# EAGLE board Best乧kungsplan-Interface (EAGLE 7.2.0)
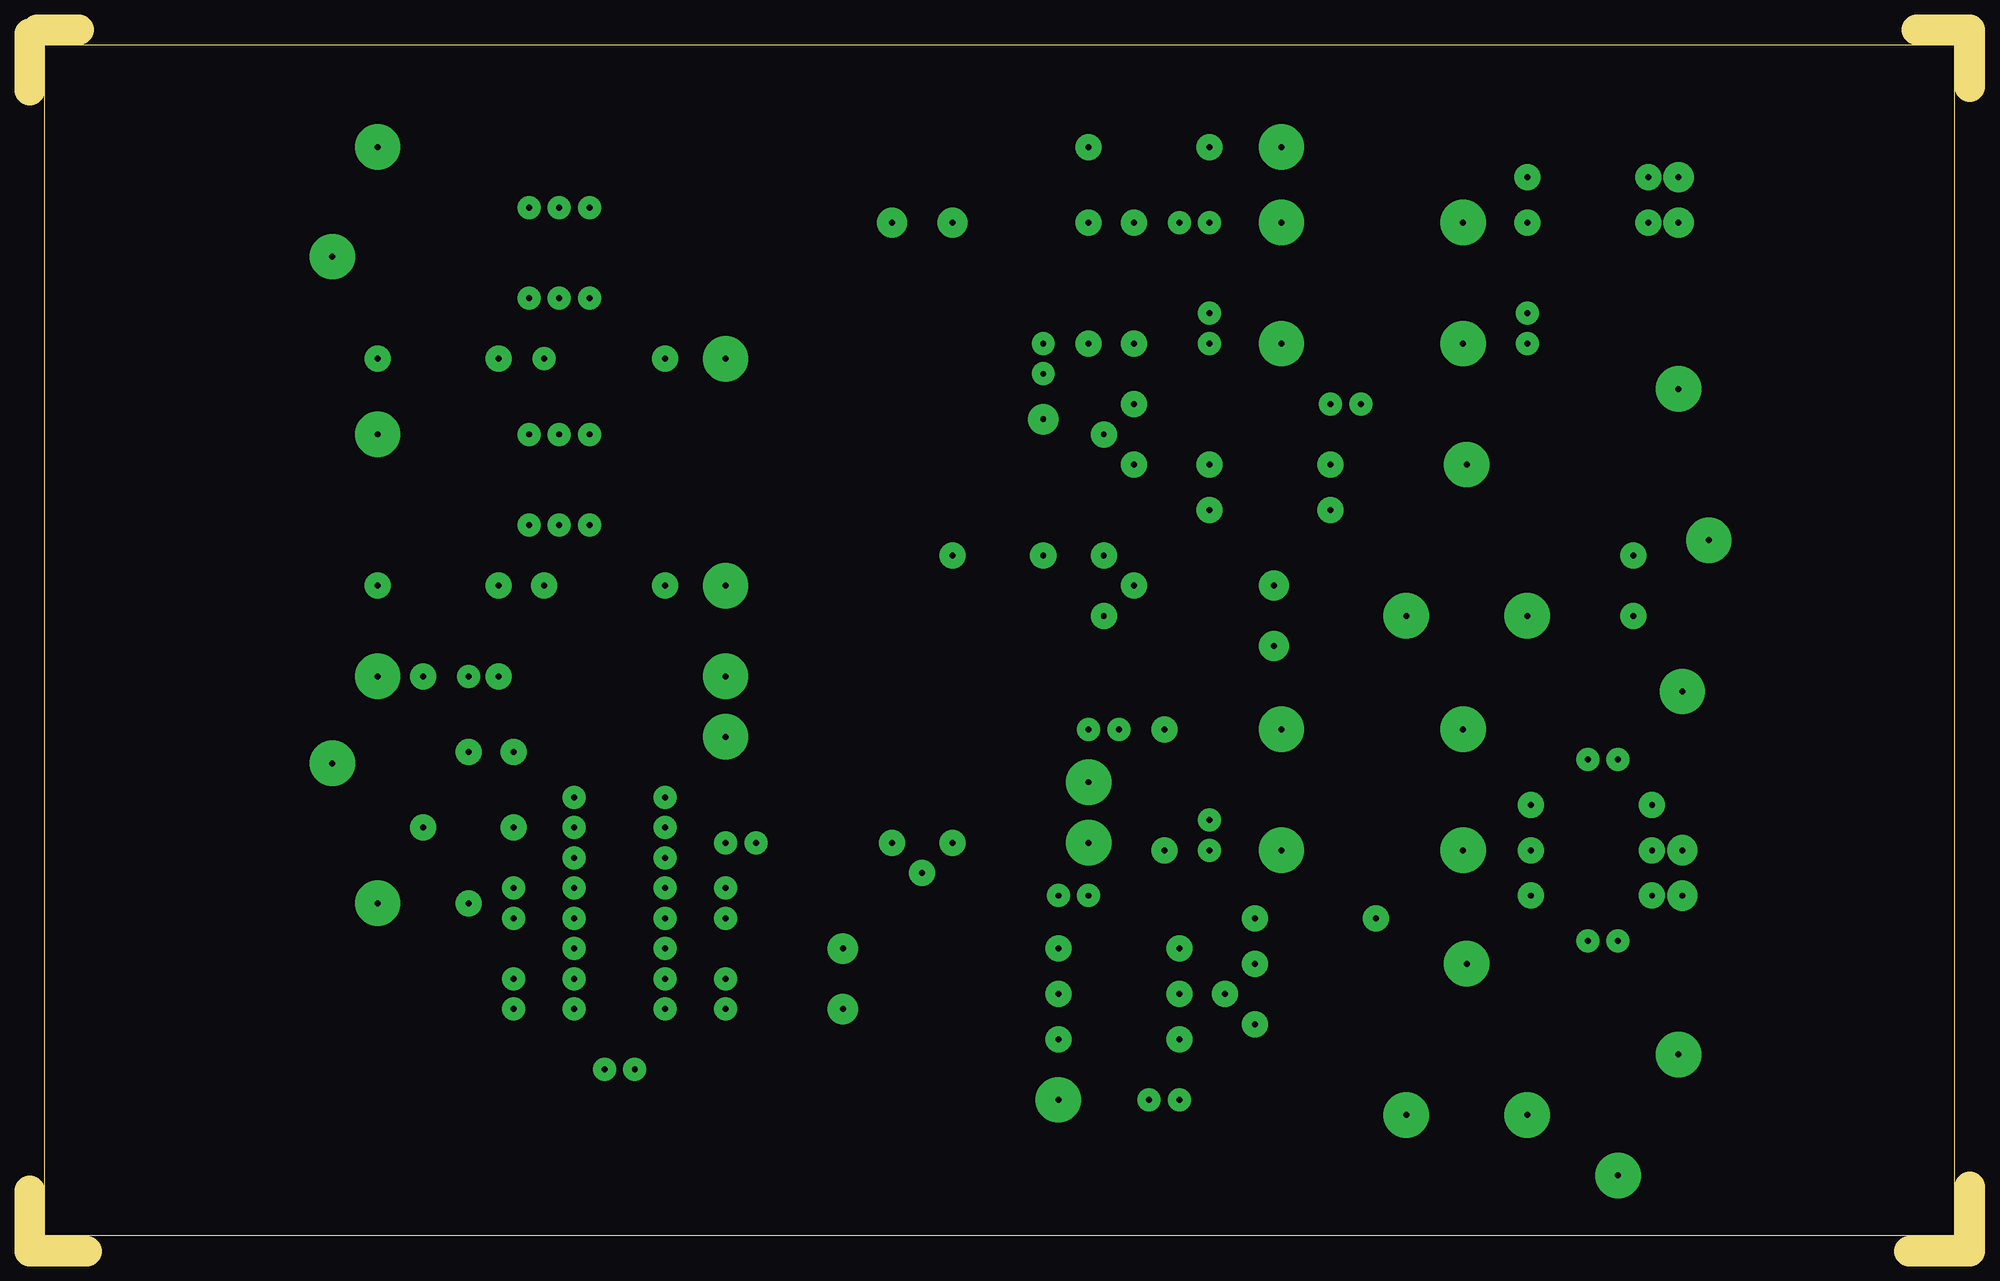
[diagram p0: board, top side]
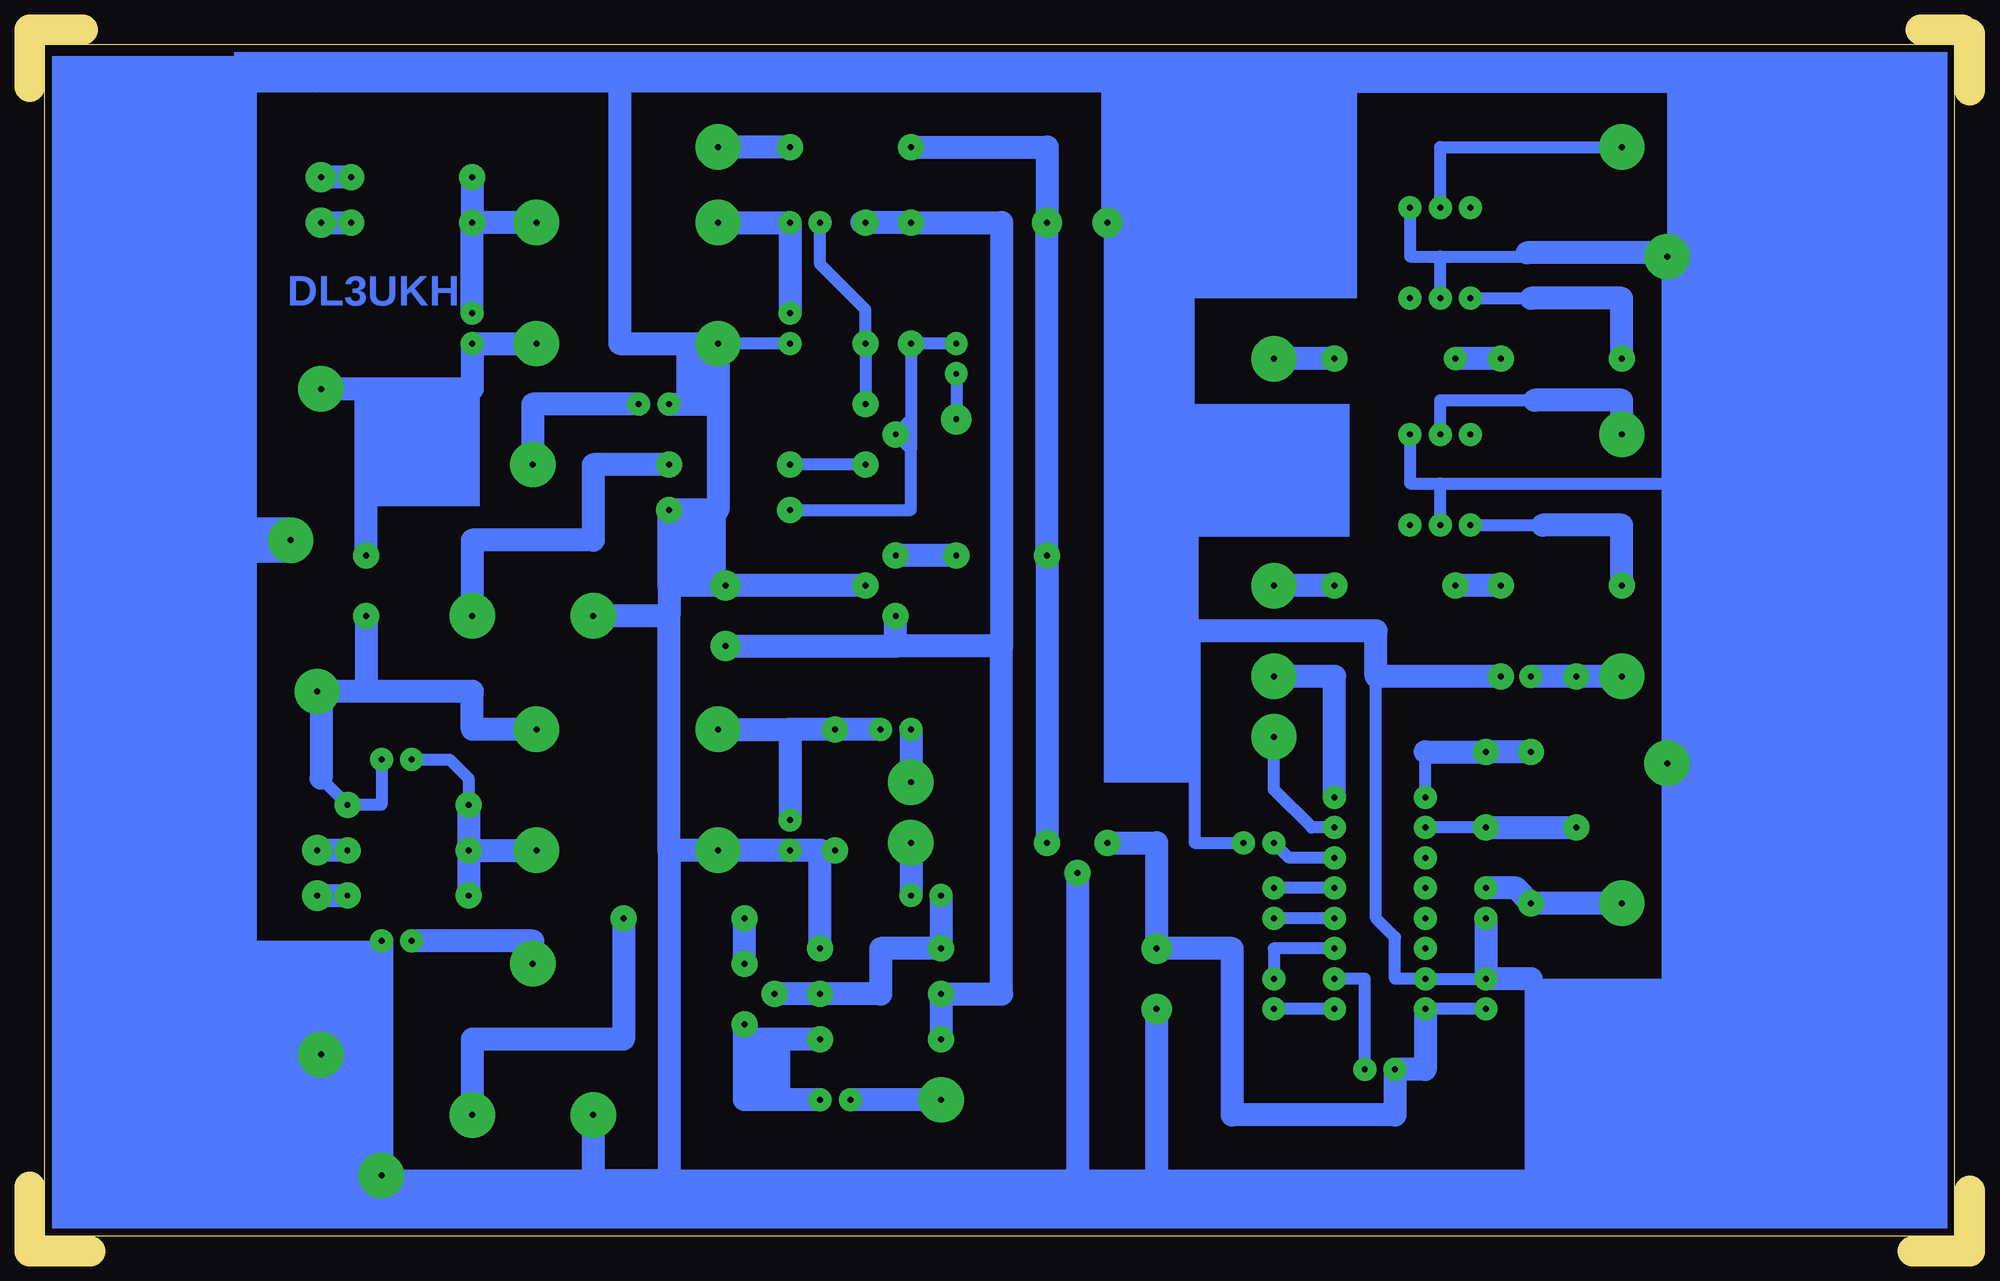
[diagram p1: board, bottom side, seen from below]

Size 162.88 x 102.55 mm. Coordinates in mm from the lower left corner, seen from the top.
Outline: 162.88,5.4 162.88,0.32
Outline: 162.88,0 157.8,0
Outline: 162.88,97.79 162.88,102.55 158.43,102.55
Outline: 0,5.08 0,0 4.76,0
Outline: 4.13,102.55 0.64,102.55
Outline: 0,97.47 0,102.23
Outline: 161.61,1.27 161.61,101.28 1.27,101.28 1.27,1.27 161.61,1.27
Copper layers (1*16): Top 0.035mm / dielectric 1.5mm / Bottom 0.035mm
Design rules "default": minimum track width 10mil, minimum drill 24mil, track to track 8mil, track to pad 8mil, pad to pad 8mil, via to via 8mil, smd to smd 8mil, copper to edge 40mil, drill to drill 8mil, minimum pad ring 10mil, minimum via ring 8mil, stop-mask expansion 4mil, vias tented up to drill 0mil, thermal gap 10mil

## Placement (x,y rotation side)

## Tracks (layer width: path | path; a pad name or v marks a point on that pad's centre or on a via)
S$1  (via drill 0.5 pad 1.93, 0.5 pad 2.18)
  Bottom 1.016: 88.9,69.85 v88.9,76.2 v85.09,76.2 | 88.9,69.85 v90.17,68.58 88.9,67.31 | 88.9,67.31 88.9,66.36 88.9,62.23 v99.06,62.23 | 88.9,69.85 88.9,67.31
S$2  (via drill 0.5 pad 3.81)
  other vias: 138.43,72.39
S$3  (via drill 0.5 pad 2.18, 0.5 pad 2.54)
  Bottom 1.93: v138.43,86.36 v135.89,86.36
S$4  (via drill 0.5 pad 1.93, 0.5 pad 2.54)
  Bottom 1.016: v85.09,73.66 v85.09,69.85
S$5  (via drill 0.5 pad 2.18, 0.5 pad 2.54)
  Bottom 1.93: v135.89,90.17 v138.43,90.17
S$6  (via drill 0.5 pad 2.18, 0.5 pad 2.54)
  Bottom 1.93: 93.03,86.36 v88.9,86.36 81.28,86.36 81.28,50.8 | v86.36,17.78 v86.36,21.59 81.28,21.59 81.28,50.8 | 81.28,50.8 90.17,50.8 | 90.17,50.8 v90.17,53.34 | v104.46,50.8 90.17,50.8
S$7
  Bottom 1.016: 138.75,97.79 145.42,97.79
S$8  (via drill 0.5 pad 1.93, 0.5 pad 3.81)
  Bottom 1.93: v105.09,86.36 v99.06,86.36 v99.06,78.74
S$9  (via drill 0.5 pad 1.93, 0.5 pad 3.81)
  Bottom 1.93: v120.65,24.13 120.65,26.04 v130.81,26.04
S$10  (via drill 0.5 pad 1.93, 0.5 pad 3.81)
  Bottom 1.93: v111.76,71.12 120.65,71.12 v120.65,66.04
S$11  (via drill 0.5 pad 1.93, 0.5 pad 2.18, 0.5 pad 3.81)
  Bottom 1.93: v105.09,43.82 99.06,43.82 | 99.06,43.82 v99.06,36.2 | 99.06,43.82 v95.25,43.82 91.76,43.82
S$12  (via drill 0.5 pad 1.93, 0.5 pad 2.18, 0.5 pad 3.81)
  Bottom 1.93: v125.73,90.17 v125.73,86.36 | v120.33,86.36 v125.73,86.36 | v125.73,78.74 v125.73,86.36
S$13  (via drill 0.5 pad 2.18)
  other vias: 92.71,86.36
S$14  (via drill 0.5 pad 2.18)
  Bottom 1.93: v102.87,24.13 v102.87,27.94
S$15  (via drill 0.5 pad 3.81)
  Bottom 1.93: 125.73,33.66 v120.33,33.66
S$16  (via drill 0.5 pad 1.93)
  other vias: 91.44,43.82
S$17  (via drill 0.5 pad 2.18)
  Bottom 1.93: v74.93,31.75 74.93,6.67
S$18  (via drill 0.5 pad 1.93, 0.5 pad 2.18)
  Bottom 1.016: v92.71,71.12 v92.71,76.2 92.71,79.06 96.52,82.87 96.52,86.04 96.84,86.36 v96.52,86.36
S$19  (via drill 0.5 pad 2.18, 0.5 pad 2.54)
  Bottom 1.93: v138.75,29.84 v136.21,29.84
S$20  (via drill 0.5 pad 2.18, 0.5 pad 2.54)
  Bottom 1.93: v136.21,33.66 v138.75,33.66
S$21  (via drill 0.5 pad 2.18)
  Bottom 1.016: v92.71,66.04 v99.06,66.04
S$22  (via drill 0.5 pad 1.93, 0.5 pad 3.81)
  Bottom 1.93: v88.9,43.82 v88.9,39.37
S$23  (via drill 0.5 pad 2.18, 0.5 pad 3.81)
  Bottom 1.93: v109.22,66.04 115.57,66.04 115.57,59.69 125.73,59.69 v125.73,53.34
S$24  (via drill 0.5 pad 1.93, 0.5 pad 2.18)
  Bottom 1.016: v40.64,35.56 v45.72,35.56
  Bottom 1.93: v40.64,35.56 v33.02,35.56
S$25  (via drill 0.5 pad 1.93, 0.5 pad 2.18)
  Bottom 1.016: v130.81,41.28 127.63,41.28 126.05,39.69 v126.05,37.47
  Bottom 1.93: v126.05,29.84 v126.05,33.66 v126.05,37.47
S$26  (via drill 0.5 pad 1.93, 0.5 pad 3.81)
  Bottom 1.016: v53.34,35.56 55.25,35.56 58.42,38.74 v58.42,43.18
S$27  (via drill 0.5 pad 1.93, 0.5 pad 2.18, 0.5 pad 3.81)
  Bottom 1.016: v133.35,41.28 133.35,37.47 v136.21,37.47 138.43,39.69 | 139.06,46.99 138.43,46.99
  Bottom 1.93: v120.33,43.82 125.73,43.82 125.73,46.99 134.62,46.99 | 134.62,46.99 138.43,46.99 138.43,39.69 | v134.62,53.34 134.62,46.99
S$28  (via drill 0.5 pad 1.93, 0.5 pad 2.18, 0.5 pad 3.81)
  Bottom 1.93: v120.33,76.2 v125.73,76.2 125.73,72.39 134.62,72.39 | 134.62,72.39 138.75,72.39 | v134.62,58.42 134.62,72.39
S$29  (via drill 0.5 pad 3.81)
  other vias: 138.75,46.99
S$30  (via drill 0.5 pad 1.93, 0.5 pad 3.81)
  Bottom 1.93: v88.9,34.29 v88.9,29.84
S$31  (via drill 0.5 pad 2.18, 0.5 pad 3.81)
  Bottom 1.93: v113.03,27.94 113.03,17.78 125.73,17.78 v125.73,11.43
S$32  (via drill 0.5 pad 1.93, 0.5 pad 2.18)
  Bottom 1.93: v86.36,29.84 v86.36,25.4 91.44,25.4 91.44,21.59 v96.52,21.59 v100.33,21.59
S$33  (via drill 0.5 pad 2.18, 0.5 pad 2.54)
  Bottom 1.93: v77.47,34.29 v77.47,58.42 v77.47,86.36 77.47,92.71 v88.9,92.71
S$34  (via drill 0.5 pad 1.93, 0.5 pad 3.81)
  Bottom 1.93: v53.34,38.1 53.34,48.26 v58.42,48.26
S$35  (via drill 0.5 pad 2.18, 0.5 pad 3.81)
  Bottom 1.016: 99.38,92.71 v99.06,92.71
  Bottom 1.93: v99.06,92.71 v105.09,92.71
S$36  (via drill 0.5 pad 2.18)
  Bottom 1.93: v85.09,58.42 v90.17,58.42
S$37  (via drill 0.5 pad 1.93)
  other vias: 58.42,20.32
S$38  (via drill 0.5 pad 1.93)
  Bottom 1.016: v50.8,15.24 50.8,22.86 v53.34,22.86
S$39  (via drill 0.5 pad 1.93, 0.5 pad 2.18, 0.5 pad 2.54)
  Bottom 1.016: 72.39,33.97 v72.39,34.29 | v40.64,20.32 v45.72,20.32
  Bottom 1.93: v45.72,20.32 45.72,15.24 v48.26,15.24 48.26,11.43 61.91,11.43 61.91,25.4 v68.26,25.4 68.26,34.29 v72.39,34.29
S$40  (via drill 0.5 pad 1.93)
  Bottom 1.016: v53.34,33.02 57.15,33.02 v58.42,34.29
S$41  (via drill 0.5 pad 1.93)
  Bottom 1.016: v53.34,30.48 v58.42,30.48
S$42  (via drill 0.5 pad 1.93)
  Bottom 1.016: v53.34,27.94 58.74,27.94
S$43  (via drill 0.5 pad 1.93)
  Bottom 1.016: v53.34,25.4 58.42,25.4 v58.42,22.86
S$44  (via drill 0.5 pad 1.93)
  other vias: 46.99,80.01
S$45  (via drill 0.5 pad 1.93)
  Bottom 1.016: v53.34,20.32 58.74,20.32
S$46  (via drill 0.5 pad 1.93, 0.5 pad 2.18)
  Bottom 1.016: v41.91,80.01 36.83,80.01
  Bottom 1.93: v29.21,74.93 29.21,80.01 36.83,80.01
S$47  (via drill 0.5 pad 1.93)
  other vias: 41.91,87.63
S$48  (via drill 0.5 pad 1.93)
  other vias: 45.72,33.02
S$49  (via drill 0.5 pad 1.93)
  other vias: 45.72,30.48
S$50  (via drill 0.5 pad 1.93)
  other vias: 45.72,27.94
S$51  (via drill 0.5 pad 1.93)
  other vias: 45.72,25.4
S$52  (via drill 0.5 pad 1.93, 0.5 pad 2.18)
  Bottom 1.016: v45.72,38.1 45.72,41.91
  Bottom 1.93: 45.72,41.91 v40.64,41.91 v36.83,41.91
S$53  (via drill 0.5 pad 1.93)
  other vias: 58.42,27.94
S$54  (via drill 0.5 pad 1.93, 0.5 pad 3.81)
  Bottom 1.016: v44.45,87.63 44.45,92.71 v29.21,92.71
S$55  (via drill 0.5 pad 3.81)
  other vias: 138.43,16.51
S$56  (via drill 0.5 pad 1.93, 0.5 pad 2.18)
  Bottom 1.93: v39.37,74.93 v43.18,74.93
S$57  (via drill 0.5 pad 1.93, 0.5 pad 2.18, 0.5 pad 3.81)
  Bottom 1.93: v40.64,30.48 38.1,30.48 v36.83,29.21 v29.21,29.21
S$58  (via drill 0.5 pad 2.18, 0.5 pad 3.81)
  Bottom 1.93: v53.34,74.93 v58.42,74.93
S$59  (via drill 0.5 pad 1.93)
  other vias: 46.99,60.96
S$60  (via drill 0.5 pad 1.93, 0.5 pad 2.18)
  Bottom 1.016: 101.6,17.78 v102.87,19.05
  Bottom 1.93: v96.52,17.78 101.6,17.78 | v96.52,12.7 102.87,12.7 v102.87,19.05
S$61  (via drill 0.5 pad 1.93, 0.5 pad 2.18)
  Bottom 1.016: v41.91,60.96 35.88,60.96
  Bottom 1.93: v29.21,55.88 29.21,60.96 35.88,60.96
S$62  (via drill 0.5 pad 1.93)
  other vias: 41.91,68.58
S$63  (via drill 0.5 pad 1.93, 0.5 pad 3.81)
  Bottom 1.016: v44.45,68.58 44.45,71.44 36.51,71.44 | 29.21,68.9 v29.21,68.58
  Bottom 1.93: 29.21,68.9 29.21,71.44 36.51,71.44
S$64
  Bottom 1.93: 25.4,83.82 37.15,83.82
S$65  (via drill 0.5 pad 2.18)
  Bottom 1.93: v39.37,55.88 v43.18,55.88
S$66  (via drill 0.5 pad 1.93, 0.5 pad 2.18, 0.5 pad 3.81)
  Bottom 1.93: v29.21,48.26 v33.02,48.26 v36.83,48.26
S$67  (via drill 0.5 pad 2.18, 0.5 pad 3.81)
  Bottom 1.93: v53.34,55.88 v58.42,55.88
S$68  (via drill 0.5 pad 1.93, 0.5 pad 3.81)
  Bottom 1.93: v86.36,12.7 v93.98,12.7
S$70  (via drill 0.5 pad 1.93, 0.5 pad 2.18, 0.5 pad 2.54, 0.5 pad 3.81)
  Bottom 1.016: v44.45,60.96 44.45,64.45 | 44.45,64.45 25.4,64.45 v25.4,40.96 | v25.4,40.96 25.4,6.35 36.83,6.35 | v72.39,86.36 72.39,97.79 | 72.39,97.79 113.35,97.79 138.43,97.79 | v95.25,33.66 96.52,33.66 | v99.06,76.2 v105.09,76.2 | v133.35,6.35 115.57,6.35 109.22,6.35 68.26,6.35 36.83,6.35 | 36.83,6.35 36.83,22.86 | v40.64,22.86 v45.72,22.86 48.26,22.86 48.26,26.35 49.85,27.94 49.85,48.26 | 65.09,52.07 65.09,34.29 v60.96,34.29 | v46.99,68.58 46.99,64.45 44.45,64.45 | v44.45,80.01 44.45,83.5 | 44.45,83.5 v25.4,83.5 v25.4,40.96 | v46.99,87.63 46.99,83.5 44.45,83.5 | 72.39,97.79 24.77,97.79
  Bottom 1.93: 105.09,71.12 v105.09,76.2 113.35,76.2 113.35,97.79 | 105.09,71.12 105.09,62.23 v109.22,62.23 109.22,55.88 | v109.22,71.12 105.09,71.12 | 109.22,55.88 109.22,53.34 | 109.22,53.34 v115.57,53.34 | 109.22,33.66 v105.09,33.66 v99.06,33.66 96.52,33.66 v96.52,25.4 | 109.22,33.66 109.22,53.34 | 109.22,33.66 109.22,6.35 | v92.71,55.88 v104.46,55.88 109.22,55.88 | v133.35,26.04 v133.35,6.35 | v115.57,11.43 115.57,6.35 | 36.83,22.86 v40.64,22.86 v40.64,27.94 | v68.26,20.32 68.26,6.35 | 65.09,52.07 49.85,52.07 49.85,48.26 v39.37,48.26
  Bottom 3.81: v140.97,59.69 145.73,59.69
(copper drawn outside any net)
  shapes: Bottom area x17

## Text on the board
Bottom: DL3UKH
Pads: AUF BESTÜCKUNGS-SEITE GESEHEN | 10n | 220µH
Dimension: K | Cevausit 1,5mm dick | alles mit 0,8mm vorgebohrt
tOrigins: 78L08 | 78L05 | Bei anderen trcvr | 1N4148 | +12V | mit 2 Stck. | K | 220µH / 10n | 470µ | PTT-Ausg. | 680 | Sound Line In | +8v | 10µ | und einzeln | 6 | trcvr Masse | als Txd / Rxd | 680 | Ausg. | Eing. | + | + | anschliessen. | 4N33 | Übertrager | Masse | ohne Brücke | 1 | 15K | 470 | COM-Port | + | 4,7n | 4,7n | anderer Ausg./Eing. | 1N4148 | Sound Masse Line In | 1,5K | An RTS | BC547c | ist als grün | K | 10µ | 10µ | mit 220µ + 10n | K | + | 6 | BC547c | 100 | CW-Ausg. | trcvr Masse | 4N33 | Poti | RX | 12K | trcvr Masse | Brücke | 1 | COM-Port | K | 250 | 1,5K | An DTR | Einstellreg. | Bei ICOM als | 1N4148 | Brücke | Ausg. | CI-V Bus | 470µ | µA78L08 | Sound Masse Line Out | An Txd | C | E | nur ein Stck. | +8v | + | 220µH / 10n | COM-Port | 10µ | B | und mit Brücke | 4,7n | trcvr Masse | + | als schwarz | 220µH | An Rxd | 1N4148 | mit 220µ + 10n | Brücke | µA78L05 | 680 | 680 | Übertrager | 100n | TX | 4,7n | Poti | 680 | 10n | Sound Line Out | CI-V | Ausg. | + | MAX232 | 680 | 10µ | 100 | 100n | 20K | + | + | 10µ | Katode | Anode | 33K | BC547c | 100n | 470µ | trcvr Masse | 16 | 1 | 100n | +8v | 1,0K | K | NF | 10µ | 500 | 100n | trcvr | Einstellreg. | + | +5v | COM-Port Masse | Aufbohren: | Einstellregler 1,2mm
